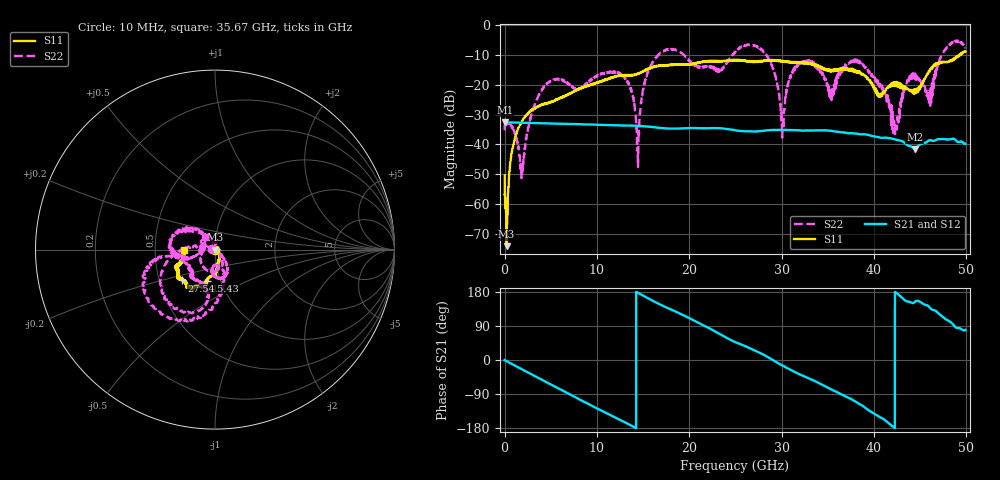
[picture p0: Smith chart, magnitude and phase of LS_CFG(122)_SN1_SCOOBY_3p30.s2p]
!Keysight Technologies,N5245B,MY58422026,A.13.80.08
!Date: Friday, March 20, 2020 00:05:31
!Correction: S11(Full 2 Port(1,2))
!S21(Full 2 Port(1,2))
!S12(Full 2 Port(1,2))
!S22(Full 2 Port(1,2))
!S2P File: Measurements: S11, S21, S12, S22:
# Hz S DB R 50.0
!freq dBS11 angS11 dBS21 angS21 dBS12 angS12 dBS22 angS22
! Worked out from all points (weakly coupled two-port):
!   4991 points, 10 MHz to 49.91 GHz, reference 50 ohm
!   highest |S21| = -32.58 dB at 30 MHz (marker M1); lowest = -41.6 dB at 44.43 GHz (marker M2)
!   lowest |S11| = -74.2 dB at 230 MHz (marker M3), VSWR 1.00, Z = 50 + j0.0193 ohm
!   |S11| at or under -10 dB: start of sweep to 49.24 GHz; 49.29295 GHz to 49.33609 GHz (43.14 MHz wide, 0.0875 % of centre)
!   |S22| runs from -51.3 to -5.1 dB; largest |S21 - S12| = 0.00024
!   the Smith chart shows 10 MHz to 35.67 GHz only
!   S11 on the Smith chart (normalised r, x): 10 MHz: 1.00, -0.01; 15.43 GHz: 0.86, -0.31; 27.54 GHz: 0.66, -0.24; 35.67 GHz: 0.71, +0.00
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1e7  -50.44 -107.8  -32.60 -0.1  -32.57 -0.2  -35.25 177.0
3e7  -57.01 -169.6  -32.58 -0.5  -32.61 -0.5  -33.76 -176.3
2.3e8  -74.16 79.8  -32.62 -3.1  -32.62 -3.2  -32.84 -166.3
2.01e9  -31.58 -41.5  -32.73 -26.1  -32.72 -26.1  -46.21 45.5
4.31e9  -26.33 -52.7  -32.94 -55.5  -32.92 -55.5  -20.40 -148.9
8.33e9  -21.15 -79.7  -33.23 -106.9  -33.23 -106.8  -20.99 -93.1
1.276e10  -16.86 -87.8  -33.65 -161.0  -33.65 -160.9  -16.79 -63.2
1.444e10  -16.31 -99.5  -33.77 177.6  -33.75 177.6  -46.21 -93.2
1.543e10  -14.95 -105.3  -34.00 164.4  -33.99 164.4  -16.55 173.3
1.665e10  -13.69 -104.9  -34.39 148.8  -34.38 148.9  -9.99 -157.4
2.496e10  -11.76 -127.4  -35.21 47.5  -35.20 47.7  -9.08 -167.8
2.754e10  -12.02 -136.7  -35.57 20.3  -35.57 20.4  -7.50 -110.3
3.011e10  -12.22 -145.4  -35.20 -14.2  -35.21 -14.0  -34.79 15.2
3.116e10  -12.40 -149.9  -35.21 -28.1  -35.22 -27.8  -15.60 140.3
3.328e10  -12.96 -158.9  -35.32 -52.2  -35.32 -51.8  -12.32 -175.3
3.567e10  -15.27 179.9  -35.61 -80.9  -35.55 -80.5  -20.87 128.0
3.816e10  -15.88 174.9  -36.41 -112.0  -36.36 -112.3  -11.57 -174.7
4.16e10  -20.36 102.1  -37.87 -166.7  -37.89 -166.8  -25.61 67.4
4.233e10  -19.47 102.7  -38.32 179.1  -38.32 179.1  -33.81 164.3
4.443e10  -22.72 48.5  -41.58 153.1  -41.64 153.3  -17.56 -12.8
4.601e10  -15.62 3.2  -38.57 139.3  -38.57 139.4  -23.30 117.0
4.991e10  -8.79 -13.9  -39.85 79.2  -39.90 78.9  -7.37 -14.7
